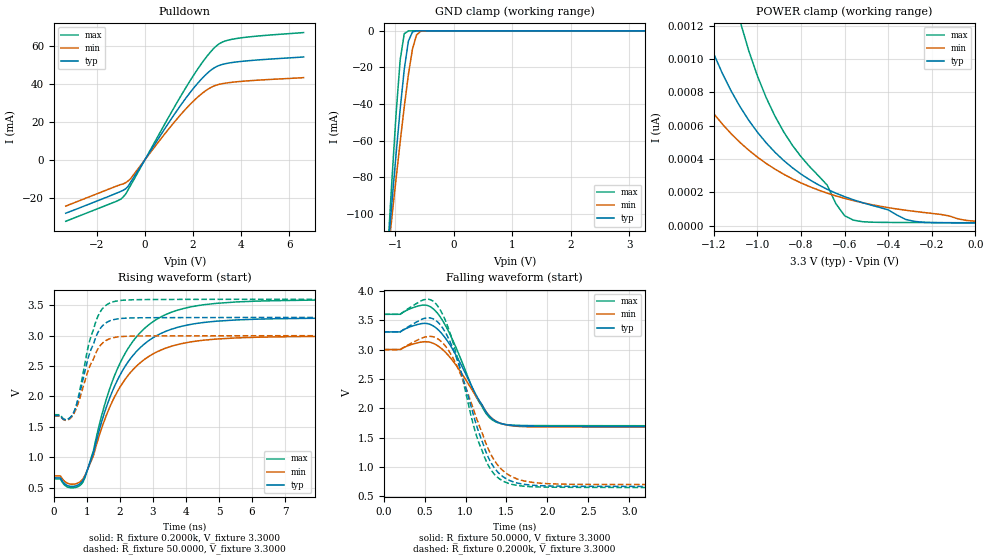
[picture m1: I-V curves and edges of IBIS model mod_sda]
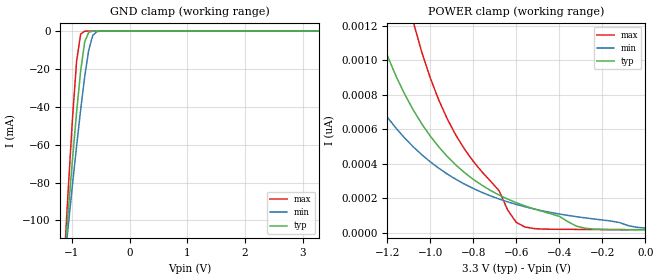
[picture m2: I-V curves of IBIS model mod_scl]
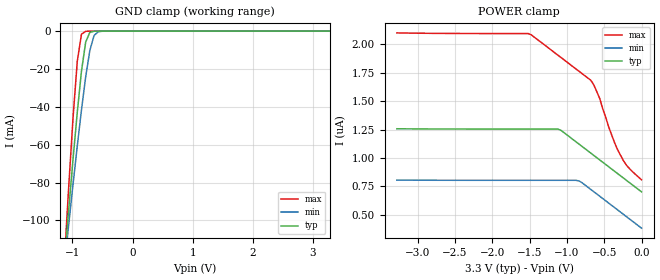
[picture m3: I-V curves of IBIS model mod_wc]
| IBIS (I/O, Buffer, Information, Specification) Model, officially
| electronic behavioral standard for Buffer structures of digital pins.
[IBIS ver]  4.0
[File name] m24512e_3d3_dfn8.ibs
[File Rev]  1.0
[Date]   26 Jan 2023
[Source]   CAD & Design Services (Catania) - STMicroelectronics
[Notes]
   (Note1)  This IBIS model includes the DFN8 package parasitic data
   (Note2)  This IBIS model has some Notes about the non-monotonicity
   of the I-V curves, but they are not indicative of problems
   inside the model;
[Disclaimer]
   Customers are solely responsible for all aspects of their
   own product designs or applications using this IBIS Model.
   STMicroelectronics assumes no liability for Custmer Designs
   and applications associated to this IBIS Model.
   In the use of this IBIS Model Customer shall not modify,
   disassemble, alter this Model in whole or in part.
   If Customers do not accept these terms, the IBIS Model
   may not be used. For any problems or modifications please
   contact STMicroelectronics (www.st.com).
[Copyright] (c) 2023 STMicroelectronics
|   Component M24512E
[Component] M24512E
[Manufacturer] STMicroelectronics
[Package]
| variable   typ   min   max
R_pkg   0.0   0.0   0.0
L_pkg   0.0H   0.0H   0.0H
C_pkg   0.0F   0.0F   0.0F
[Pin]   signal_name   model_name   R_pin   L_pin   C_pin
1   NC   NC   0.0   0.0   0.0
2   NC   NC   0.0   0.0   0.0
3   NC   NC   0.0   0.0   0.0
4   VSS   GND   0.0   0.0   0.0
5   SDA   mod_sda   0.0   0.0   0.0
6   SCL   mod_scl   0.0   0.0   0.0
7   WC   mod_wc   0.0   0.0   0.0
8   VCC   POWER   0.0   0.0   0.0
[Package Model]  182694_DFN8   | also called 182694_MLP_2x3
[Define Package Model]  182694_DFN8
[Manufacturer]  STMicroelectronics
[OEM]  STMicroelectronics
[Description]  8 pin DFN8 2x3
[Number Of Pins]  8
[Pin Numbers]
|Pin Num   Terminal Name
1   | net1
2   | net2
3   | net3
4   | net4_GND
5   | net5
6   | net6
7   | net7
8   | net8_VDD
[Model Data]
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[End Model Data]
[End Package Model]
| Models and submodels in the file (3): mod_sda (I/O_open_drain), mod_scl (Input), mod_wc (Input)
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|   Model mod_sda
[Model]   mod_sda
Model_type I/O_open_drain
Polarity   Inverting
Enable   Active-High
Vinl   =   0.990V
Vinh   =   2.310V
Vmeas  =   1.650V
Cref   =   30pF
Rref   =   500
Vref   =   3.300V
C_comp   2.548pF   2.320pF   2.655pF
[Model Spec]
Vinl   0.990V  0.900V  1.080V  | <- for Vcc = 3.3V, 3.0V, 3.6V
Vinh   2.310V  2.100V  2.520V  | <- for Vcc = 3.3V, 3.0V, 3.6V
Vmeas  1.650V  1.500V  1.800V  | <- for Vcc = 3.3V, 3.0V, 3.6V
[Temperature Range]  25.0000   85.0000   -40.0000
[Voltage Range]   3.3000V   3.0000V   3.6000V
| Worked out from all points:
|   slope of the pulldown table from 0 to 0.495 V, typ, clamps not added: 50.2 ohm
|   GND clamp passes 1 mA (typ) near -0.72 V on its own axis
|   rising waveform, R_fixture 0.2000k, V_fixture 3.3000: 20-80 % time 1.3ns typ, 1.31ns min, 1.29ns max; typ from 0.663 V to 3.29 V
|   rising waveform, R_fixture 50.0000, V_fixture 3.3000: 20-80 % time 507ps typ, 519ps min, 487ps max; typ from 1.69 V to 3.3 V
|   falling waveform, R_fixture 50.0000, V_fixture 3.3000: 20-80 % time 367ps typ, 369ps min, 355ps max; typ from 3.3 V to 1.69 V
|   falling waveform, R_fixture 0.2000k, V_fixture 3.3000: 20-80 % time 360ps typ, 382ps min, 343ps max; typ from 3.3 V to 0.664 V
[Pulldown]
|Voltage   I(typ)   I(min)   I(max)
-3.3V     -28.28mA   -24.52mA   -32.53mA
-1.2V     -17.76mA   -14.02mA   -22.03mA
-900mV    -16.13mA   -12.74mA   -19.57mA
-700mV    -14.04mA   -11.24mA   -15.82mA
-600mV    -11.94mA   -10.06mA   -13.59mA
900mV     17.78mA    14.8mA     20.54mA
1.8V      34.11mA    28.11mA    40.04mA
2.5V      44.45mA    36.13mA    53.22mA
3V        49.23mA    39.41mA    60.28mA
3.3V      50.47mA    40.25mA    62.41mA
3.9V      51.65mA    41.15mA    64.06mA
6.6V      54.14mA    43.24mA    67.02mA
[GND_clamp]
|Voltage   I(typ)   I(min)   I(max)
-3.3V     -1.01A     -814.9mA   -1.404A
-1.13V    -120.1mA   -122.5mA   -118.8mA
-1.06V    -93.42mA   -101.5mA   -81.03mA
-990mV    -67.49mA   -80.83mA   -45.6mA
-920mV    -42.94mA   -60.76mA   -15.96mA
-850mV    -21.15mA   -41.63mA   -1.606mA
-780mV    -5.768mA   -24.18mA   -63.74uA
-710mV    -616.4uA   -10.08mA   -4.14uA
-640mV    -45.34uA   -2.266mA   -227.5nA
-570mV    -3.307uA   -288.2uA   -7.345nA
3.28V     15.71pA    85.37pA    15.34pA
[POWER_clamp]
|Voltage   I(typ)   I(min)   I(max)
-3.28V    8.276uA    4.441uA    14.63uA
-1.44V    2.157nA    1.226nA    5.11nA
-1.4V     1.906nA    1.108nA    4.359nA
-1.24V    1.164nA    741.3pA    2.31nA
-1.16V    911.1pA    607.7pA    1.684nA
-1.08V    714pA      499.1pA    1.229nA
-960mV    496.8pA    373.1pA    768.5pA
-880mV    391.1pA    308.5pA    563.5pA
-680mV    217.9pA    194.7pA    242.9pA
-600mV    173.5pA    163.3pA    59.05pA
-280mV    25.23pA    85.37pA    18.25pA
0V        15.81pA    26.21pA    16.88pA
[Ramp]
| variable   typ   min   max
dV/dt_r  0.9667/0.5182n   0.7932/0.5320n   1.1394/0.4984n
dV/dt_f  0.9667/0.3847n   0.7934/0.3893n   1.1396/0.3661n
R_load = 50.0000
[Rising Waveform]
R_fixture= 0.2000k
V_fixture= 3.3000
V_fixture_min= 3.0000
V_fixture_max= 3.6000
|time   V(typ)   V(min)   V(max)
0s        663.4mV    695.7mV    645.6mV
510ps     523.8mV    560.1mV    500.1mV
880ps     619.9mV    646.7mV    592.8mV
1.2ns     1.072V     1.029V     1.112V
1.6ns     1.841V     1.704V     1.976V
1.98ns    2.328V     2.133V     2.52V
2.52ns    2.751V     2.508V     2.992V
3.2ns     3.025V     2.753V     3.295V
4.92ns    3.237V     2.944V     3.53V
10ns      3.292V     2.992V     3.592V
[Rising Waveform]
R_fixture= 50.0000
V_fixture= 3.3000
V_fixture_min= 3.0000
V_fixture_max= 3.6000
|time   V(typ)   V(min)   V(max)
0s        1.689V     1.677V     1.701V
200ps     1.689V     1.677V     1.701V
360ps     1.616V     1.608V     1.621V
590ps     1.723V     1.702V     1.723V
750ps     1.977V     1.909V     2.009V
1.05ns    2.651V     2.443V     2.842V
1.27ns    2.974V     2.713V     3.228V
1.47ns    3.16V      2.875V     3.441V
1.75ns    3.254V     2.959V     3.548V
10ns      3.3V       2.999V     3.599V
[Falling Waveform]
R_fixture= 50.0000
V_fixture= 3.3000
V_fixture_min= 3.0000
V_fixture_max= 3.6000
|time   V(typ)   V(min)   V(max)
0s        3.3V       3V         3.6V
200ps     3.3V       3V         3.6V
470ps     3.443V     3.13V      3.756V
610ps     3.397V     3.102V     3.686V
830ps     3.033V     2.833V     3.2V
1.11ns    2.276V     2.242V     2.256V
1.23ns    1.986V     1.988V     1.958V
1.33ns    1.816V     1.822V     1.8V
1.49ns    1.722V     1.72V      1.725V
10ns      1.689V     1.678V     1.701V
[Falling Waveform]
R_fixture= 0.2000k
V_fixture= 3.3000
V_fixture_min= 3.0000
V_fixture_max= 3.6000
|time   V(typ)   V(min)   V(max)
0s        3.3V       3V         3.6V
530ps     3.54V      3.222V     3.858V
660ps     3.467V     3.181V     3.739V
880ps     2.892V     2.765V     2.962V
1.1ns     1.863V     1.964V     1.692V
1.24ns    1.291V     1.436V     1.141V
1.38ns    936.5mV    1.058V     838.8mV
1.58ns    750mV      826.8mV    701.4mV
2.32ns    673.1mV    706.7mV    655mV
10ns      664.4mV    696.8mV    646.3mV
|   Model mod_scl
[Model]   mod_scl
Model_type Input
Vinl   =   0.990V
Vinh   =   2.310V
C_comp   1.062pF   1.014pF   1.112pF
[Model Spec]
Vinl   0.990V  0.900V  1.080V  | <- for Vcc = 3.3V, 3.0V, 3.6V
Vinh   2.310V  2.100V  2.520V  | <- for Vcc = 3.3V, 3.0V, 3.6V
[Temperature Range]  25.0000   85.0000   -40.0000
[Voltage Range]   3.3000V   3.0000V   3.6000V
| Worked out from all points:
|   GND clamp passes 1 mA (typ) near -0.72 V on its own axis
[GND_clamp]
|Voltage   I(typ)   I(min)   I(max)
-3.3V     -1.01A     -814.9mA   -1.404A
-1.13V    -120.1mA   -122.5mA   -118.8mA
-1.06V    -93.42mA   -101.5mA   -81.03mA
-990mV    -67.49mA   -80.83mA   -45.6mA
-920mV    -42.94mA   -60.76mA   -15.96mA
-850mV    -21.15mA   -41.63mA   -1.606mA
-780mV    -5.768mA   -24.18mA   -63.74uA
-710mV    -616.4uA   -10.08mA   -4.14uA
-640mV    -45.34uA   -2.266mA   -227.5nA
-570mV    -3.307uA   -288.2uA   -7.345nA
3.28V     15.71pA    85.37pA    15.34pA
[POWER_clamp]
|Voltage   I(typ)   I(min)   I(max)
-3.28V    8.276uA    4.441uA    14.63uA
-1.44V    2.157nA    1.226nA    5.11nA
-1.4V     1.906nA    1.108nA    4.359nA
-1.24V    1.164nA    741.3pA    2.31nA
-1.16V    911.1pA    607.7pA    1.684nA
-1.08V    714pA      499.1pA    1.229nA
-960mV    496.8pA    373.1pA    768.5pA
-880mV    391.1pA    308.5pA    563.5pA
-680mV    217.9pA    194.7pA    242.9pA
-600mV    173.5pA    163.3pA    59.05pA
-280mV    25.23pA    85.37pA    18.25pA
0V        15.81pA    26.21pA    16.88pA
|   Model mod_wc
[Model]   mod_wc
Model_type Input
Vinl   =   0.990V
Vinh   =   2.310V
C_comp   1.062pF   1.014pF   1.112pF
[Model Spec]
Vinl   0.990V  0.900V  1.080V  | <- for Vcc = 3.3V, 3.0V, 3.6V
Vinh   2.310V  2.100V  2.520V  | <- for Vcc = 3.3V, 3.0V, 3.6V
[Temperature Range]  25.0000   85.0000   -40.0000
[Voltage Range]   3.3000V   3.0000V   3.6000V
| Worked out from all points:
|   GND clamp passes 1 mA (typ) near -0.72 V on its own axis
[GND_clamp]
|Voltage   I(typ)   I(min)   I(max)
-3.3V     -1.01A     -814.9mA   -1.404A
-1.13V    -120.1mA   -122.5mA   -118.8mA
-1.06V    -93.42mA   -101.5mA   -81.03mA
-990mV    -67.49mA   -80.83mA   -45.6mA
-920mV    -42.94mA   -60.76mA   -15.97mA
-850mV    -21.15mA   -41.63mA   -1.616mA
-780mV    -5.773mA   -24.18mA   -77.12uA
-710mV    -625.1uA   -10.09mA   -18.69uA
-640mV    -55.88uA   -2.271mA   -13.28uA
-570mV    -13.75uA   -295.5uA   -10.92uA
3.28V     30.9uA     28.12uA    35.04uA
[POWER_clamp]
|Voltage   I(typ)   I(min)   I(max)
-3.28V    1.257uA    805.9nA    2.098uA
-1.52V    1.254uA    804.3nA    2.092uA
-1.48V    1.254uA    804.3nA    2.082uA
-1.12V    1.254uA    804.3nA    1.902uA
-840mV    1.123uA    799nA      1.762uA
-680mV    1.043uA    724.3nA    1.682uA
-640mV    1.023uA    704.3nA    1.642uA
-560mV    983nA      664.3nA    1.522uA
-440mV    923nA      604.3nA    1.272uA
-320mV    863nA      544.3nA    1.072uA
-200mV    803nA      484.3nA    935nA
0V        703nA      384.3nA    808.8nA
